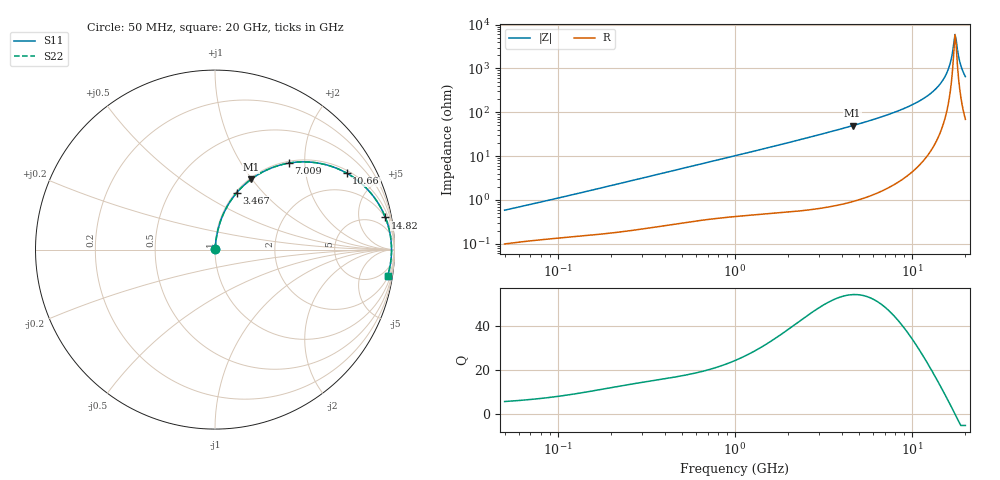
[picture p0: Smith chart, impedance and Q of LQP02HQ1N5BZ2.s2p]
!Murata Part Number: LQP02HQ1N5BZ2
!These Parameters are Measured in Series Mode Connection
!  o--[Z]--o
!Port1  Port2
!  o-------o
!Freq. Start=50[MHz] Stop=20[GHz], 401[Steps]
# Hz S RI R 50
!Freq.(Hz) S11(Real) S11(Imag) S21(Real) S21(Imag) S12(Real) S12(Imag) S22(Real) S22(Imag)
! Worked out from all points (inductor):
!   401 points, 50 MHz to 20 GHz, reference 50 ohm
!   read as one part in series: L = 1.79 nH near 51.52 MHz
!   highest Q = 54.1 at 4.608 GHz (marker M1), where L = 1.71 nH
!   self-resonance near 17.48 GHz
!   S11 on the Smith chart (normalised r, x): 50 MHz: 1.00, +0.01; 3.467 GHz: 1.01, +0.72; 7.009 GHz: 1.03, +1.67; 10.66 GHz: 1.11, +3.38; 14.82 GHz: 2, +10; 20 GHz: 2, -13
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5e7  0.00102 0.00574  0.999 -0.00574  0.999 -0.00574  0.00102 0.00574
1.364002e8  0.00172 0.0146  0.9983 -0.0146  0.9983 -0.0146  0.00172 0.0146
3.721004e8  0.00396 0.0386  0.996 -0.0386  0.996 -0.0386  0.00396 0.0386
1e9  0.0142 0.0997  0.9858 -0.0997  0.9858 -0.0997  0.0142 0.0997
2.728004e9  0.0773 0.2565  0.9227 -0.2565  0.9227 -0.2565  0.0773 0.2565
3.466789e9  0.1198 0.3151  0.8802 -0.3151  0.8802 -0.3151  0.1198 0.3151
4.608136e9  0.2008 0.3915  0.7992 -0.3915  0.7992 -0.3915  0.2008 0.3915
7.009217e9  0.4114 0.4819  0.5886 -0.4819  0.5886 -0.4819  0.4114 0.4819
7.442007e9  0.452 0.4871  0.548 -0.4871  0.548 -0.4871  0.452 0.4871
9.041845e9  0.5996 0.4773  0.4004 -0.4773  0.4004 -0.4773  0.5996 0.4773
1.066139e10  0.7339 0.4259  0.2661 -0.4259  0.2661 -0.4259  0.7339 0.4259
1.295331e10  0.8783 0.3024  0.1217 -0.3024  0.1217 -0.3024  0.8783 0.3024
1.482269e10  0.9493 0.179  0.0507 -0.179  0.0507 -0.179  0.9493 0.179
1.597544e10  0.9729 0.1008  0.0271 -0.1008  0.0271 -0.1008  0.9729 0.1008
1.646126e10  0.9787 0.0683  0.0213 -0.0683  0.0213 -0.0683  0.9787 0.0683
1.721783e10  0.9833 0.0188  0.0167 -0.0188  0.0167 -0.0188  0.9833 0.0188
1.747767e10  0.9837 0.00227  0.0163 -0.00227  0.0163 -0.00227  0.9837 0.00227
1.774144e10  0.9835 -0.0143  0.0165 0.0143  0.0165 0.0143  0.9835 -0.0143
1.800918e10  0.9828 -0.0309  0.0172 0.0309  0.0172 0.0309  0.9828 -0.0309
1.855685e10  0.9797 -0.0639  0.0203 0.0639  0.0203 0.0639  0.9797 -0.0639
1.912117e10  0.9744 -0.0965  0.0256 0.0965  0.0256 0.0965  0.9744 -0.0965
2e10  0.9624 -0.1443  0.0376 0.1443  0.0376 0.1443  0.9624 -0.1443
